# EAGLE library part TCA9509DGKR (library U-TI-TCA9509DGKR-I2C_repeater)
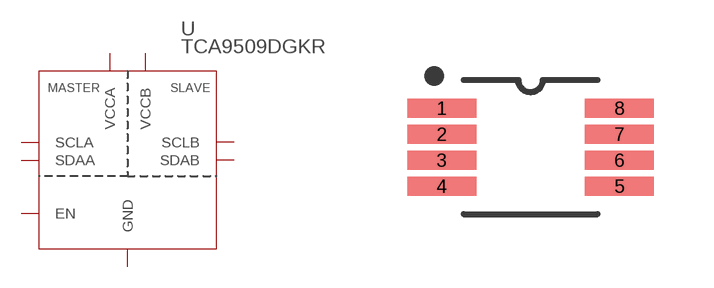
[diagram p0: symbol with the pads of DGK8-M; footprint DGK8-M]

Designator prefix U

## TCA9509DGKRDGK8-M (MANUFACTURER_PART_NUMBER: TCA9509DGKR; VENDOR: Texas Instruments)  [DGK8-M]
1  VCCA  pwr
2  SCLA
3  SDAA
4  GND  pwr
5  EN  in
6  SDAB
7  SCLB
8  VCCB  pwr

## Footprint DGK8-M (pad centres in mm)
smd 1.727 x 0.483: 1 -2.223,0.975; 2 -2.223,0.325; 3 -2.223,-0.325; 4 -2.223,-0.975; 5 2.223,-0.975; 6 2.223,-0.325; 7 2.223,0.325; 8 2.223,0.975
